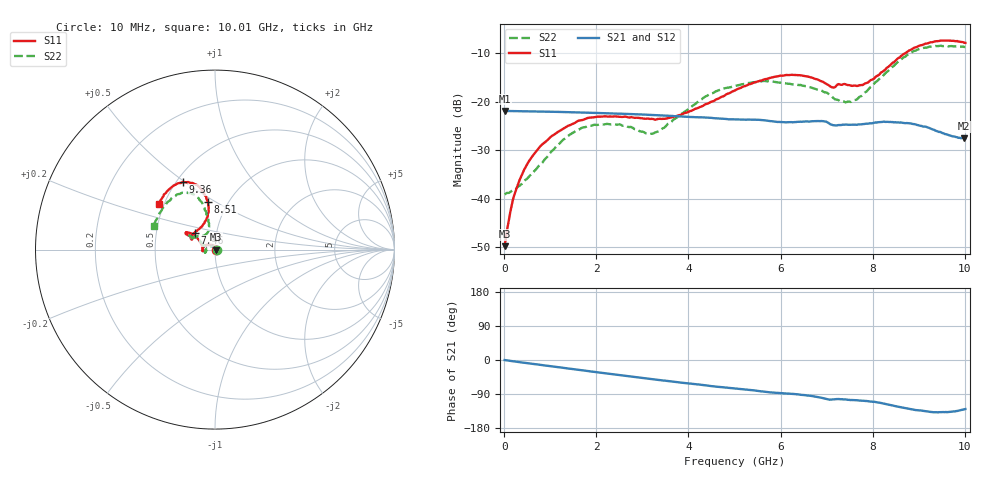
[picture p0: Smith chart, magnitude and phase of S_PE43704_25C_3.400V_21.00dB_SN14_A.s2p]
! Device ID: PE43704
! Dir: z:\PE43704\PE43704_Char_1_20130516\PE43704\AMB\3p400V\21p00dB
! Serial: 14
! Insertion: A
! Impedance: 50 ohm
! Temp: Amb
! VDD: 3.400V
! Attenuation Step: 21.00dB
! IDD: 1.140731e-01mA
#  Hz  S  RI  R  50
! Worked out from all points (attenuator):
!   401 points, 10 MHz to 10.01 GHz, reference 50 ohm
!   highest |S21| = -21.93 dB at 10 MHz (marker M1); lowest = -27.5 dB at 9.985 GHz (marker M2)
!   lowest |S11| = -49.7 dB at 10 MHz (marker M3), VSWR 1.01, Z = 50.3 + j0.0484 ohm
!   |S11| at or under -10 dB: start of sweep to 8.718 GHz
!   |S22| runs from -39.1 to -8.5 dB; largest |S21 - S12| = 0.00079
!   S11 on the Smith chart (normalised r, x): 10 MHz: 1.01, +0.00; 7.46 GHz: 0.78, +0.15; 8.51 GHz: 0.81, +0.46; 9.36 GHz: 0.54, +0.49; 10.01 GHz: 0.47, +0.28
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1e7  0.00322 0.000481  0.0801 -0.00024  0.0801 -0.000182  0.0111 0.000318
1.6e8  0.00285 0.00789  0.0797 -0.00386  0.0797 -0.00382  0.0105 0.00585
2.35e8  0.00141 0.0114  0.0795 -0.0056  0.0795 -0.00551  0.00896 0.00871
5.35e8  -0.00711 0.0232  0.0784 -0.0122  0.0784 -0.0122  0.000121 0.0168
1.035e9  -0.0325 0.0299  0.0752 -0.0228  0.0752 -0.0227  -0.0253 0.0179
1.685e9  -0.0624 0.0155  0.0686 -0.0353  0.0686 -0.0352  -0.0536 -0.00154
2.26e9  -0.07 -0.00165  0.0611 -0.0445  0.0612 -0.0445  -0.0566 -0.0157
3.135e9  -0.0663 -0.0058  0.0477 -0.0554  0.0476 -0.0555  -0.0469 -0.00134
3.36e9  -0.0664 -0.000276  0.0437 -0.0575  0.0437 -0.0574  -0.0489 0.00773
4.41e9  -0.084 0.0441  0.0262 -0.0633  0.0264 -0.0632  -0.0969 0.0619
5.01e9  -0.108 0.0725  0.0171 -0.0634  0.0171 -0.0633  -0.1264 0.0705
5.96e9  -0.1557 0.0958  0.0032 -0.0616  0.00344 -0.0616  -0.1406 0.0694
6.685e9  -0.1556 0.0822  -0.0058 -0.0625  -0.00588 -0.0623  -0.1215 0.0659
7.11e9  -0.1249 0.0642  -0.0143 -0.0561  -0.0143 -0.056  -0.0827 0.0764
7.46e9  -0.114 0.0939  -0.0151 -0.0557  -0.0149 -0.0561  -0.0517 0.0857
7.835e9  -0.0677 0.1377  -0.0184 -0.056  -0.0182 -0.0562  -0.0339 0.1201
8.36e9  -0.0359 0.2297  -0.0295 -0.0541  -0.029 -0.0545  -0.0485 0.2067
8.51e9  -0.0385 0.2647  -0.0326 -0.0516  -0.0323 -0.0521  -0.0613 0.2389
8.935e9  -0.0889 0.3505  -0.039 -0.043  -0.0387 -0.0427  -0.1271 0.3098
9.36e9  -0.1791 0.3763  -0.0372 -0.0336  -0.0374 -0.0339  -0.2152 0.3047
9.985e9  -0.3073 0.2597  -0.027 -0.0321  -0.0276 -0.0324  -0.3367 0.1383
1.001e10  -0.3124 0.2515  -0.0267 -0.0324  -0.0272 -0.0327  -0.3406 0.1296
